| NXP Semiconductors
| Logic Products Group
| IBIS model of 74LVC2G126
| DUAL BUS BUFFER/LINE DRIVER; 3-STATE
|[Packages]:
|[Package1]: TSSOP8 (DP) 8-pins package
|[Package2]: VSSOP8 (DC) 8-pins package
|[Package3]: XSON8 (GT) 8-pins Package
|[Package4]: XSON8 (GF) 8-pins Package
|[Package5]: XSON8U (GD) 8-pins package
|[Package6]: XSON8 (GN) 8-pins Package
|[Package7]: XSON8 (GS) 8-pins Package
|[Package8]: XQFN8 (GM) 8-pins package
[IBIS Ver]   3.2
[File Name]   lvc2g126.ibs
[File Rev]   1.2
[Date]   14-Jan-2015
[Source]   File created from simulations by LPG
   NXP Semiconductors Nijmegen
[Notes]   V1.2   Ibis model.
| Revision History
| Version Date   Author/ Description
|   Editor
| 1.0   July   2003 RM   Initial Version
| 1.1   December 2004 RRV   Added XSON package
| 1.2   December 2011 GY   Updated models,added GN,GS package
| Remarks:
| 1. The Power Clamp curves have been omitted since there is no power clamp
|   diode.
| 2. Non-monotonic sections below 0V in pulldown and pullup curves have been
|   removed (if any).
[Disclaimer]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
[Copyright]
   (C) Copyright 2015 NXP Semiconductors
   All rights reserved
|   Info for  TSSOP8 (DP) 8-pins package
[Component]   74LVC2G126_DP
[Manufacturer]   NXP Semiconductors
[Package]
|   Typ   Min   Max
R_pkg   7.796E-02   6.927E-02   8.662E-02
L_pkg   1.612E-09   1.470E-09   1.752E-09
C_pkg   3.647E-13   3.408E-13   3.889E-13
[Pin] signal_name   model_name   R_pin   L_pin   C_pin
   1   1OE   LVC2G126_CTRLIN 8.661E-02 1.752E-09 3.411E-13
   2   1A   LVC2G126_IN 6.930E-02 1.472E-09 3.889E-13
   3   2Y   LVC2G126_AHTRISTN 6.932E-02 1.475E-09 3.883E-13
   4   GND   GND 8.662E-02 1.752E-09 3.410E-13
   5   2A   LVC2G126_IN 8.662E-02 1.751E-09 3.408E-13
   6   1Y   LVC2G126_AHTRISTN 6.930E-02 1.472E-09 3.880E-13
   7   2OE   LVC2G126_CTRLIN 6.927E-02 1.470E-09 3.883E-13
   8   VCC   POWER 8.662E-02 1.750E-09 3.409E-13
|   Info for  VSSOP8 (DC) 8-pins package
[Component]   74LVC2G126_DC
[Manufacturer]   NXP Semiconductors
[Package]
|   Typ   Min   Max
R_pkg   8.321E-02   8.287E-02   8.533E-02
L_pkg   1.585E-09   1.544E-09   1.824E-09
C_pkg   3.093E-13   2.504E-13   5.556E-13
[Pin] signal_name   model_name   R_pin   L_pin   C_pin
   1   1OE   LVC2G126_CTRLIN 8.295E-02 1.560E-09 2.505E-13
   2   1A   LVC2G126_IN 8.290E-02 1.546E-09 2.924E-13
   3   2Y   LVC2G126_AHTRISTN 8.288E-02 1.546E-09 2.896E-13
   4   GND   GND 8.533E-02 1.824E-09 5.556E-13
   5   2A   LVC2G126_IN 8.295E-02 1.560E-09 2.504E-13
   6   1Y   LVC2G126_AHTRISTN 8.287E-02 1.544E-09 2.920E-13
   7   2OE   LVC2G126_CTRLIN 8.289E-02 1.545E-09 2.920E-13
   8   VCC   POWER 8.293E-02 1.559E-09 2.516E-13
|   Info for  XSON8 (GT) 8-pins Package
[Component]   74LVC2G126_GT
[Manufacturer]   NXP Semiconductors
[Package]
|   Typ   Min   Max
R_pkg   4.241E-02   3.477E-02   5.228E-02
L_pkg   5.404E-10   4.419E-10   6.673E-10
C_pkg   1.195E-13   1.144E-13   1.275E-13
[Pin] signal_name   model_name   R_pin   L_pin   C_pin
   1   1OE   LVC2G126_CTRLIN 4.701E-02 6.002E-10 1.203E-13
   2   1A   LVC2G126_IN 3.559E-02 4.525E-10 1.154E-13
   3   2Y   LVC2G126_AHTRISTN 3.478E-02 4.421E-10 1.144E-13
   4   GND   GND 5.228E-02 6.673E-10 1.275E-13
   5   2A   LVC2G126_IN 5.228E-02 6.672E-10 1.275E-13
   6   1Y   LVC2G126_AHTRISTN 3.477E-02 4.419E-10 1.145E-13
   7   2OE   LVC2G126_CTRLIN 3.558E-02 4.523E-10 1.154E-13
   8   VCC   POWER 4.701E-02 5.996E-10 1.211E-13
|   Info for  XSON8 (GF) 8-pins Package
[Component]   74LVC2G126_GF
[Manufacturer]   NXP Semiconductors
[Package]
|   Typ   Min   Max
R_pkg   3.673E-02   3.526E-02   3.882E-02
L_pkg   4.676E-10   4.489E-10   4.948E-10
C_pkg   1.130E-13   1.067E-13   1.165E-13
[Pin] signal_name   model_name   R_pin   L_pin   C_pin
   1   1OE   LVC2G126_CTRLIN 3.526E-02 4.496E-10 1.067E-13
   2   1A   LVC2G126_IN 3.655E-02 4.648E-10 1.165E-13
   3   2Y   LVC2G126_AHTRISTN 3.631E-02 4.617E-10 1.162E-13
   4   GND   GND 3.882E-02 4.948E-10 1.119E-13
   5   2A   LVC2G126_IN 3.882E-02 4.946E-10 1.120E-13
   6   1Y   LVC2G126_AHTRISTN 3.630E-02 4.615E-10 1.163E-13
   7   2OE   LVC2G126_CTRLIN 3.654E-02 4.646E-10 1.165E-13
   8   VCC   POWER 3.526E-02 4.489E-10 1.076E-13
|   Info for  XSON8U (GD) 8-pins package
[Component]   74LVC2G126_GD
[Manufacturer]   NXP Semiconductors
[Package]
|   Typ   Min   Max
R_pkg   7.877E-02   7.876E-02   7.877E-02
L_pkg   1.209E-09   1.209E-09   1.209E-09
C_pkg   1.410E-13   1.367E-13   1.439E-13
[Pin] signal_name   model_name   R_pin   L_pin   C_pin
   1   1OE   LVC2G126_CTRLIN 7.876E-02 1.209E-09 1.426E-13
   2   1A   LVC2G126_IN 7.877E-02 1.209E-09 1.439E-13
   3   2Y   LVC2G126_AHTRISTN 7.877E-02 1.209E-09 1.435E-13
   4   GND   GND 7.876E-02 1.209E-09 1.367E-13
   5   2A   LVC2G126_IN 7.876E-02 1.209E-09 1.369E-13
   6   1Y   LVC2G126_AHTRISTN 7.877E-02 1.209E-09 1.435E-13
   7   2OE   LVC2G126_CTRLIN 7.877E-02 1.209E-09 1.435E-13
   8   VCC   POWER 7.876E-02 1.209E-09 1.372E-13
|   Info for  XSON8 (GN) 8-pins Package
[Component]   74LVC2G126_GN
[Manufacturer]   NXP Semiconductors
[Package]
|   Typ   Min   Max
R_pkg   4.574E-02   4.573E-02   4.574E-02
L_pkg   5.846E-10   5.845E-10   5.846E-10
C_pkg   1.431E-13   1.301E-13   1.562E-13
[Pin] signal_name   model_name   R_pin   L_pin   C_pin
   1   1OE   LVC2G126_CTRLIN 4.573E-02 5.846E-10 1.302E-13
   2   1A   LVC2G126_IN 4.574E-02 5.845E-10 1.562E-13
   3   2Y   LVC2G126_AHTRISTN 4.574E-02 5.845E-10 1.560E-13
   4   GND   GND 4.574E-02 5.846E-10 1.301E-13
   5   2A   LVC2G126_IN 4.574E-02 5.846E-10 1.301E-13
   6   1Y   LVC2G126_AHTRISTN 4.574E-02 5.845E-10 1.561E-13
   7   2OE   LVC2G126_CTRLIN 4.574E-02 5.845E-10 1.562E-13
   8   VCC   POWER 4.574E-02 5.846E-10 1.302E-13
|   Info for  XSON8 (GS) 8-pins Package
[Component]   74LVC2G126_GS
[Manufacturer]   NXP Semiconductors
[Package]
|   Typ   Min   Max
R_pkg   5.159E-02   5.158E-02   5.159E-02
L_pkg   6.596E-10   6.595E-10   6.596E-10
C_pkg   1.499E-13   1.368E-13   1.630E-13
[Pin] signal_name   model_name   R_pin   L_pin   C_pin
   1   1OE   LVC2G126_CTRLIN 5.158E-02 6.596E-10 1.369E-13
   2   1A   LVC2G126_IN 5.159E-02 6.595E-10 1.630E-13
   3   2Y   LVC2G126_AHTRISTN 5.159E-02 6.595E-10 1.628E-13
   4   GND   GND 5.159E-02 6.596E-10 1.369E-13
   5   2A   LVC2G126_IN 5.159E-02 6.596E-10 1.368E-13
   6   1Y   LVC2G126_AHTRISTN 5.159E-02 6.595E-10 1.628E-13
   7   2OE   LVC2G126_CTRLIN 5.159E-02 6.595E-10 1.629E-13
   8   VCC   POWER 5.159E-02 6.596E-10 1.370E-13
|   Info for  XQFN8 (GM) 8-pins package
[Component]   74LVC2G126_GM
[Manufacturer]   NXP Semiconductors
[Package]
|   Typ   Min   Max
R_pkg   5.536E-02   5.534E-02   5.540E-02
L_pkg   8.470E-10   8.457E-10   8.490E-10
C_pkg   1.446E-13   1.411E-13   1.462E-13
[Pin] signal_name   model_name   R_pin   L_pin   C_pin
   1   2OE   LVC2G126_CTRLIN 5.534E-02 8.461E-10 1.454E-13
   2   1Y   LVC2G126_AHTRISTN 5.534E-02 8.458E-10 1.453E-13
   3   2A   LVC2G126_IN 5.539E-02 8.490E-10 1.460E-13
   4   GND   GND 5.534E-02 8.459E-10 1.414E-13
   5   2Y   LVC2G126_AHTRISTN 5.539E-02 8.490E-10 1.461E-13
   6   1A   LVC2G126_IN 5.534E-02 8.457E-10 1.453E-13
   7   1OE   LVC2G126_CTRLIN 5.540E-02 8.490E-10 1.462E-13
   8   VCC   POWER 5.534E-02 8.459E-10 1.411E-13
[Model Selector]   LVC2G126_CTRLIN
LVC_XGCTRLIN_33   3.3V-Vcc input model
LVC_XGCTRLIN_50   5.0V-Vcc input model
LVC_XGCTRLIN_25   2.5V-Vcc input model
LVC_XGCTRLIN_18   1.8V-Vcc input model
[Model Selector]   LVC2G126_AHTRISTN
LVC_XGAHTRISTN_33   3.3V-Vcc tristate non-inverting output model (active high)
LVC_XGAHTRISTN_50   5.0V-Vcc tristate non-inverting output model (active high)
LVC_XGAHTRISTN_25   2.5V-Vcc tristate non-inverting output model (active high)
LVC_XGAHTRISTN_18   1.8V-Vcc tristate non-inverting output model (active high)
[Model Selector]   LVC2G126_IN
LVC_XGIN_33   3.3V-Vcc input model
LVC_XGIN_50   5.0V-Vcc input model
LVC_XGIN_25   2.5V-Vcc input model
LVC_XGIN_18   1.8V-Vcc input model
| Models and submodels in the file (12): LVC_XGCTRLIN_33 (Input), LVC_XGCTRLIN_50 (Input), LVC_XGCTRLIN_25 (Input), LVC_XGCTRLIN_18 (Input), LVC_XGIN_33 (Input), LVC_XGIN_50 (Input), LVC_XGIN_25 (Input), LVC_XGIN_18 (Input), LVC_XGAHTRISTN_33 (3-state), LVC_XGAHTRISTN_50 (3-state), LVC_XGAHTRISTN_25 (3-state), LVC_XGAHTRISTN_18 (3-state)
